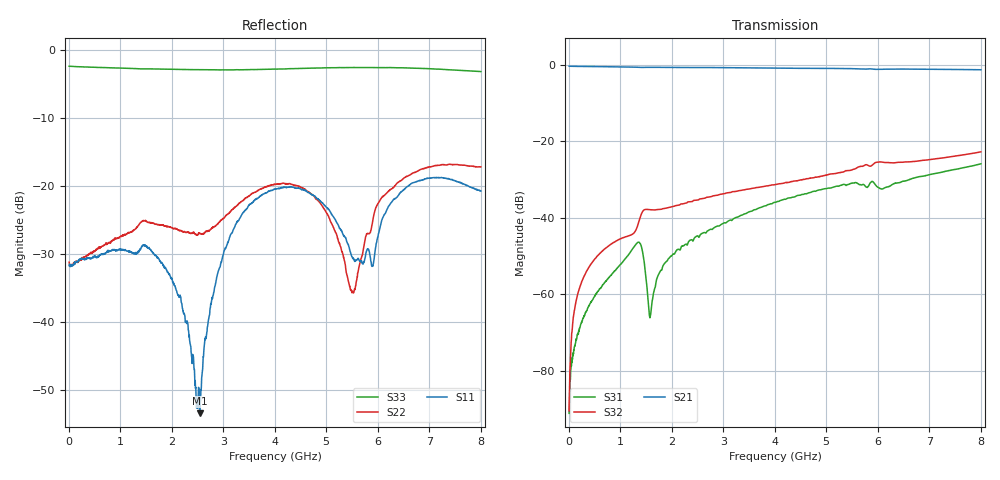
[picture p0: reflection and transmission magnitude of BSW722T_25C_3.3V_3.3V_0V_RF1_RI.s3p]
! Product: BSW722T
! Temp: 25C
! VDD: 3.300
! Control_Hi: 3.300
! Control_Lo: 0.000
! Logic State: RF1
! Port 1: RFC
! Port 2: RF1
! Port 3: RF2
! V1 = 3.30
! V2 = 0.00
! V3 = 0.00
! V4 = 0.00
# Hz S  RI  R 50
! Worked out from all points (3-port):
!   1601 points, 5 MHz to 8.005 GHz, reference 50 ohm
!   strongest paths, dB at 5 MHz, 2.005 GHz, 4.005 GHz, 6.005 GHz, 8.005 GHz:
!     S21: -0.3, -0.6, -0.8, -1.1, -1.2
!     S32: -90.5, -37.1, -31.3, -25.4, -22.7
!     S31: -91.1, -49.7, -35.9, -32.0, -25.8
!   lowest |S11| = -53.4 dB at 2.54 GHz (marker M1), VSWR 1.00, Z = 49.8 + j0.117 ohm
!   |S11| at or under -10 dB: start of sweep to end of sweep
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5000000  0.0259 -0.000931  0.9674 -0.0102  -1.53e-05 -1.42e-05
         0.9671 -0.00961  0.0274 -0.00134  -4.49e-06 2.27e-05
         -1.19e-05 -2.51e-05  1.32e-05 2.67e-05  -0.7544 0.00678
2.75e8  0.0243 -0.0158  0.8632 -0.4176  -4.62e-05 0.000494
        0.8633 -0.4176  0.0248 -0.0164  0.000579 0.0015
        -3.81e-05 0.000485  0.000586 0.00148  -0.6738 0.3196
1.085e9  -0.0278 -0.019  -0.1787 -0.9274  0.00282 0.000412
         -0.1788 -0.9274  -0.0283 -0.033  0.00557 0.000621
         0.00283 0.00041  0.00557 0.000627  0.1108 0.7209
1.585e9  -0.0292 0.0175  -0.78 -0.5147  -3.16e-05 0.000524
         -0.78 -0.5146  -0.0536 0.000945  0.0102 -0.00771
         -2.62e-05 0.000529  0.0102 -0.00772  0.5849 0.422
2.54e9  -0.00178 0.00117  -0.5418 0.7534  0.00153 -0.00558
        -0.5418 0.7536  -0.0302 0.0327  -0.00911 -0.0152
        0.00154 -0.00557  -0.00911 -0.0152  0.4175 -0.5756
4.005e9  0.0242 0.0921  0.9 -0.1443  -0.0136 0.00858
         0.9001 -0.1443  0.0448 0.092  -0.012 0.0244
         -0.0136 0.00858  -0.012 0.0244  -0.7 0.1647
4.915e9  0.0707 -0.0257  -0.0396 -0.9043  0.0122 0.0203
         -0.0399 -0.9045  0.0701 -0.0132  0.0261 0.024
         0.0122 0.0203  0.0259 0.0239  0.0607 0.7304
5.85e9  -0.0235 0.0201  -0.8925 -0.0202  0.0244 -0.0145
        -0.8924 -0.0203  -0.0196 0.0405  0.0374 -0.0293
        0.0245 -0.0143  0.0373 -0.0293  0.7343 0.0806
6.885e9  0.1095 -0.0148  0.0634 0.8804  -0.0165 -0.031
         0.0631 0.8801  0.1267 0.0431  -0.0369 -0.0432
         -0.0166 -0.0311  -0.0368 -0.0432  0.1096 -0.7178
8.005e9  -0.0873 -0.027  0.8232 -0.277  -0.0375 0.0346
         0.8226 -0.2773  0.0879 -0.1059  -0.0527 0.051
         -0.0375 0.0346  -0.0526 0.0509  -0.6868 0.0533
